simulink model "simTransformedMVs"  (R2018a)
settings: Solver=ode15s  StartTime=0.0  StopTime=tsim  MaxStep=theta/100  RelTol=1e-3
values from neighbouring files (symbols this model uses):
  c0 = 10    [BaseCase.m]    (also in TransformedMVs.m)
  dc = 0*c0    (= 0)    [BaseCase.m]    (also in TransformedMVs.m = 1)
  dM = 0*M0    (= 0)    [BaseCase.m]    (also in TransformedMVs.m)
  dq = 0.1*q0    (= 1)    [BaseCase.m]    (also in TransformedMVs.m = 0)
  du = [0;0.5]    [BaseCase.m]    (also in TransformedMVs.m)
  Kc_c = 1/k.c*tau.c/(tauC.c+theta)    [BaseCase.m]    (also in TransformedMVs.m)
  Kc_M = 1/k.M/(tauC.M+theta)    [BaseCase.m]    (also in TransformedMVs.m)
  M0 = 1    [BaseCase.m]    (also in TransformedMVs.m = 100; H2P_Turbine_driven.m = param(22); runTD.m = 7.56; H2P_Boiler_driven.m = param(22))
  p = [c1; c2; tau02]    [BaseCase.m]    (also in TransformedMVs.m; Main.m = [N, Fc0, rhoc, rhoh,U,A,cpc,cph]; Main_OL.m = [N, Fc0, rhoc, rhoh,U,A,cpc,cph]; runTestCalcBlk.m = [N, Fc0, rhoc, rhoh,U,A,cpc,cph])
  q0 = 10    [BaseCase.m]    (also in TransformedMVs.m)
  tauI_c = min(tau.c,4*(tauC.c+theta))    [BaseCase.m]    (also in TransformedMVs.m)
  tauI_M = 4*(tauC.M+theta)    [BaseCase.m]    (also in TransformedMVs.m)
  theta = 0    [BaseCase.m]    (also in TransformedMVs.m = 30; Main.m = 40; Main_OL.m = 40; runTransf.m = [40;60;60])
  tsim = 150    [BaseCase.m]    (also in TransformedMVs.m = 500; runTD.m = 300; runBD.m = 300; runFP.m = 300)
  tstep_c = 10    [BaseCase.m]    (also in TransformedMVs.m)
  tstep_d = 100    [BaseCase.m]    (also in TransformedMVs.m)
  tstep_M = 20    [BaseCase.m]    (also in TransformedMVs.m)
  u0 = [q10;q20]    [BaseCase.m]    (also in TransformedMVs.m; runH2Psim.m = [mG0;zV0;mP0;mB0;mA0]; calcblock.m = p(2); testfun.m = 5)
  v1_0 = q10+q20-q0    (= 0)    [BaseCase.m]    (also in TransformedMVs.m)
  v2_0 = tau02/M0*(q10*c1+q20*c2)+(1-tau02/taur)*c0    (= 10)    [BaseCase.m]    (also in TransformedMVs.m)
  x0 = [M0;c0]    [BaseCase.m]    (also in TransformedMVs.m; runTD.m = [TE0;TD0;TSh0;MD0; MSh0;w0;TA0;0;0;0;0;0;0;0;0;0]; runBD.m = [TE0;TD0;TSh0;MD0; MSh0;w0;TA0;0;0;0;0;0;0;0;0;0]; runFP.m = [TE0;TD0;TSh0;MD0; MSh0;w0;TA0;0;0;0;0;0;0;0])
undefined symbols (not defined in the file or in its folder): CalcBlock, model
libraries: simulink x2

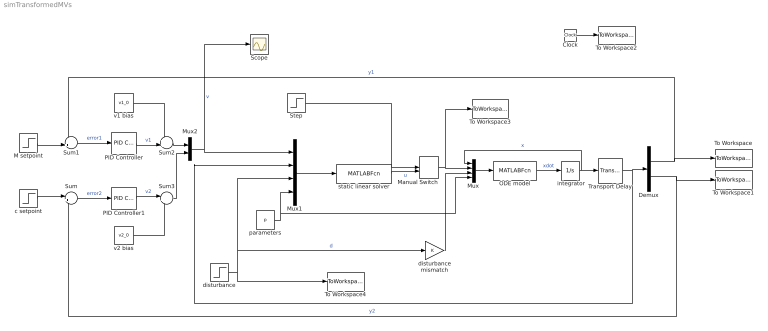
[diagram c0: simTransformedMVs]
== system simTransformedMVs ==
  " integrator" : Integrator  InitialCondition=x0
  Clock : Clock
  Demux : Demux  Outputs=2
  M setpoint : Step  Time=tstep_M  Before=M0  After=M0+dM  SampleTime=0
  Manual Switch : ManualSwitch  CurrentSetting=0
  Mux : Mux
  Mux1 : Mux
  Mux2 : Mux  Inputs=2
  ODE model : MATLABFcn  MATLABFcn=model(u(1:2), u(3:4),u(5),u(6:8))  OutputDimensions=2
  PID Controller : simulink/Continuous/PID Controller  Controller=PI  TimeDomain=Continuous-time  SampleTime=-1  IntegratorMethod=Forward Euler  FilterMethod=Forward Euler  Form=Ideal  UseFilter=on  ControllerParametersSource=internal  P=Kc_M  I=1/tauI_M  D=0  N=100  InitialConditionSource=internal  InitialConditionForIntegrator=0  InitialConditionForFilter=0  ExternalReset=none  LimitOutput=off  UpperSaturationLimit=inf  LowerSaturationLimit=-inf  LinearizeAsGain=on  AntiWindupMode=none  Kb=1  TrackingMode=off  Kt=1  PParamMin=[]  PParamMax=[]  IParamMin=[]  IParamMax=[]  DParamMin=[]  DParamMax=[]  NParamMin=[]  NParamMax=[]  KbParamMin=[]  KbParamMax=[]  KtParamMin=[]  KtParamMax=[]  POutMin=[]  POutMax=[]  IOutMin=[]  IOutMax=[]  DOutMin=[]  DOutMax=[]  NOutMin=[]  NOutMax=[]  KbOutMin=[]  KbOutMax=[]  KtOutMin=[]  KtOutMax=[]  IntegratorOutMin=[]  IntegratorOutMax=[]  FilterOutMin=[]  FilterOutMax=[]  SumOutMin=[]  SumOutMax=[]  SumI1OutMin=[]  SumI1OutMax=[]  SumI2OutMin=[]  SumI2OutMax=[]  SumI3OutMin=[]  SumI3OutMax=[]  SumDOutMin=[]  SumDOutMax=[]  SaturationOutMin=[]  SaturationOutMax=[]  IntegratorContinuousStateAttributes=''  IntegratorStateMustResolveToSignalObject=off  IntegratorRTWStateStorageClass=Auto  FilterContinuousStateAttributes=''  FilterStateMustResolveToSignalObject=off  FilterRTWStateStorageClass=Auto  DifferentiatorICPrevScaledInput=0  DifferentiatorOutMin=[]  DifferentiatorOutMax=[]  FilterDiffOutCoefMin=[]  FilterDiffOutCoefMax=[]  SumDenOutMin=[]  SumDenOutMax=[]  SumNumOutMin=[]  SumNumOutMax=[]  ReciprocalOutMin=[]  ReciprocalOutMax=[]  DivideOutMin=[]  DivideOutMax=[]  TunerSelectOption=Transfer Function Based (PID Tuner App)
  PID Controller1 : simulink/Continuous/PID Controller  Controller=PI  TimeDomain=Continuous-time  SampleTime=-1  IntegratorMethod=Forward Euler  FilterMethod=Forward Euler  Form=Ideal  UseFilter=on  ControllerParametersSource=internal  P=Kc_c  I=1/tauI_c  D=0  N=100  InitialConditionSource=internal  InitialConditionForIntegrator=0  InitialConditionForFilter=0  ExternalReset=none  LimitOutput=off  UpperSaturationLimit=inf  LowerSaturationLimit=-inf  LinearizeAsGain=on  AntiWindupMode=none  Kb=1  TrackingMode=off  Kt=1  PParamMin=[]  PParamMax=[]  IParamMin=[]  IParamMax=[]  DParamMin=[]  DParamMax=[]  NParamMin=[]  NParamMax=[]  KbParamMin=[]  KbParamMax=[]  KtParamMin=[]  KtParamMax=[]  POutMin=[]  POutMax=[]  IOutMin=[]  IOutMax=[]  DOutMin=[]  DOutMax=[]  NOutMin=[]  NOutMax=[]  KbOutMin=[]  KbOutMax=[]  KtOutMin=[]  KtOutMax=[]  IntegratorOutMin=[]  IntegratorOutMax=[]  FilterOutMin=[]  FilterOutMax=[]  SumOutMin=[]  SumOutMax=[]  SumI1OutMin=[]  SumI1OutMax=[]  SumI2OutMin=[]  SumI2OutMax=[]  SumI3OutMin=[]  SumI3OutMax=[]  SumDOutMin=[]  SumDOutMax=[]  SaturationOutMin=[]  SaturationOutMax=[]  IntegratorContinuousStateAttributes=''  IntegratorStateMustResolveToSignalObject=off  IntegratorRTWStateStorageClass=Auto  FilterContinuousStateAttributes=''  FilterStateMustResolveToSignalObject=off  FilterRTWStateStorageClass=Auto  DifferentiatorICPrevScaledInput=0  DifferentiatorOutMin=[]  DifferentiatorOutMax=[]  FilterDiffOutCoefMin=[]  FilterDiffOutCoefMax=[]  SumDenOutMin=[]  SumDenOutMax=[]  SumNumOutMin=[]  SumNumOutMax=[]  ReciprocalOutMin=[]  ReciprocalOutMax=[]  DivideOutMin=[]  DivideOutMax=[]  TunerSelectOption=Transfer Function Based (PID Tuner App)
  Scope : Scope
  Step : Step  Time=tsim/10  Before=u0  After=u0+du  SampleTime=0
  Sum : Sum  Inputs=|+-
  Sum1 : Sum  Inputs=-+|
  Sum2 : Sum  Inputs=++|
  Sum3 : Sum  Inputs=|++
  To Workspace : ToWorkspace  VariableName=M  SampleTime=-1
  To Workspace1 : ToWorkspace  VariableName=c  SampleTime=-1
  To Workspace2 : ToWorkspace  VariableName=time  SampleTime=-1
  To Workspace3 : ToWorkspace  VariableName=u  SampleTime=-1
  To Workspace4 : ToWorkspace  VariableName=d  SampleTime=-1
  Transport Delay : TransportDelay  DelayTime=theta  InitialOutput=[M0;c0]  BufferSize=2048
  c setpoint : Step  Time=tstep_c  Before=c0  After=c0+dc  SampleTime=0
  disturbance : Step  Time=tstep_d  Before=q0  After=q0+dq  SampleTime=0
  disturbance mismatch : Gain
  parameters : Constant  Value=p
  static linear solver : MATLABFcn  MATLABFcn=CalcBlock(u(1:2),u(3:4),u(5),u(6:8))  OutputDimensions=2
  v1 bias : Constant  Value=v1_0
  v2 bias : Constant  Value=v2_0
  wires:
  ODE model/1 -> " integrator"/1  "xdot"
  Demux/1 -> Sum1/1, To Workspace/1  "y1"
  Mux/1 -> ODE model/1
  Clock/1 -> To Workspace2/1
  Sum/1 -> PID Controller1/1  "error2"
  c setpoint/1 -> Sum/1
  Sum1/1 -> PID Controller/1  "error1"
  M setpoint/1 -> Sum1/2
  static linear solver/1 -> Manual Switch/2  "u"
  PID Controller/1 -> Sum2/2  "v1"
  PID Controller1/1 -> Sum3/1  "v2"
  v1 bias/1 -> Sum2/1
  v2 bias/1 -> Sum3/2
  Mux1/1 -> static linear solver/1
  Sum2/1 -> Mux2/1
  Sum3/1 -> Mux2/2
  Demux/2 -> To Workspace1/1, Sum/2  "y2"
  disturbance/1 -> To Workspace4/1, Mux1/3, disturbance mismatch/1  "d"
  " integrator"/1 -> Mux/1, Transport Delay/1  "x"
  Step/1 -> Manual Switch/1
  Manual Switch/1 -> To Workspace3/1, Mux/2
  disturbance mismatch/1 -> Mux/3
  Mux2/1 -> Scope/1, Mux1/1  "v"
  parameters/1 -> Mux/4, Mux1/4
  Transport Delay/1 -> Demux/1, Mux1/2
